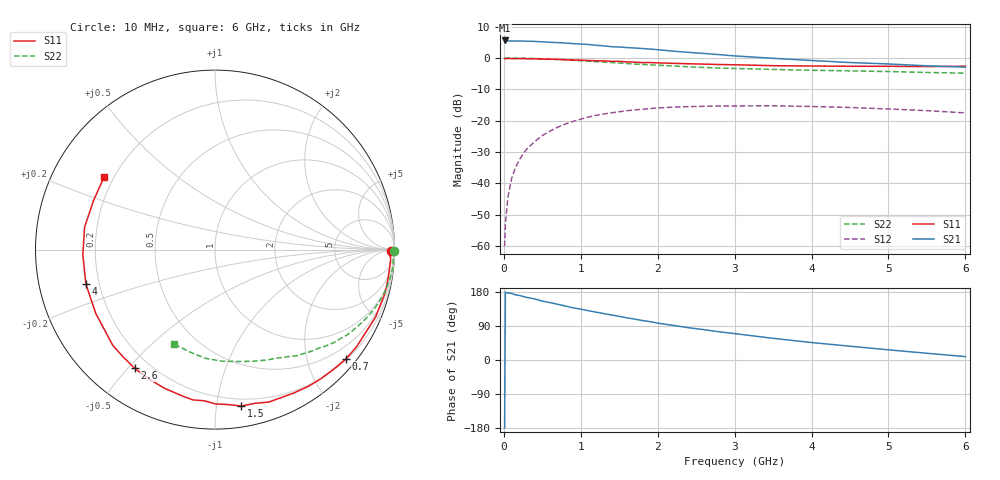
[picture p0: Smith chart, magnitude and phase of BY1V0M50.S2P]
! SIEMENS Small Signal Semiconductors
! BFY420
! Si NPN RF SIEGET Grounded Emitter Transistor in MICRO-X
! VCE = 1 V  IC = 0.5 mA
! Common Emitter S-Parameters:  October  1996
# GHz  S  MA  R  50
!  f  S11  S21  S12  S22
! GHz  MAG  ANG  MAG  ANG  MAG  ANG  MAG  ANG
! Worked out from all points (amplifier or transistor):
!   36 points, 10 MHz to 6 GHz, reference 50 ohm
!   highest |S21| = 5.6 dB at 10 MHz (marker M1)
!   |S21| within 3 dB of that: start of sweep to 2.022 GHz
!   unconditionally stable (mu >= 1): 4.728 GHz to end of sweep
!   at 250 MHz: K = 0.02, MSG = 18.0 dB, |S12| = -30.6 dB
!   at 1.4 GHz: K = 0.22, MSG = 10.5 dB, |S12| = -17.5 dB
!   at 6 GHz: K = 1.37, MAG = 3.7 dB, |S12| = -17.5 dB
!   S11 on the Smith chart (normalised r, x): 10 MHz: 80, -43; 700 MHz: 0.22, -2.75; 1.5 GHz: 0.15, -1.17; 2.6 GHz: 0.14, -0.52; 4 GHz: 0.15, -0.13; 6 GHz: 0.16, +0.29
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0.01  0.9808 -0.6  1.903 -179.2  0.001 101.0  0.9995 -0.4
0.02  0.9704 -1.3  1.888 178.8  0.0022 79.4  0.9999 -0.6
0.05  0.98 -2.8  1.874 177.1  0.0057 87.3  0.9986 -1.5
0.1  0.9783 -5.9  1.865 175.7  0.0119 88.1  0.9941 -3.0
0.15  0.9773 -8.5  1.863 172.0  0.0177 83.5  0.9951 -4.6
0.2  0.9777 -11.6  1.865 170.5  0.0237 82.2  0.9954 -6.0
0.3  0.9731 -17.3  1.849 165.2  0.0355 78.9  0.9887 -9.1
0.4  0.9701 -23.0  1.838 161.2  0.0465 75.0  0.9808 -12.1
0.5  0.9583 -28.7  1.806 155.4  0.0581 71.2  0.971 -15.0
0.7  0.9507 -39.7  1.76 147.0  0.0787 64.1  0.9463 -20.5
0.9  0.9304 -50.6  1.695 137.7  0.0977 56.8  0.9176 -25.7
1.1  0.912 -61.0  1.64 130.1  0.1142 50.3  0.8886 -30.7
1.5  0.884 -80.4  1.495 115.2  0.1391 37.9  0.8309 -39.3
1.8  0.8443 -94.1  1.416 104.1  0.1521 30.1  0.7894 -44.9
2.2  0.8219 -110.2  1.285 91.4  0.1647 20.3  0.7485 -52.1
2.6  0.7983 -124.1  1.18 80.1  0.1695 12.6  0.7074 -58.2
3  0.7799 -137.0  1.079 69.6  0.1721 5.5  0.6814 -64.4
3.5  0.7536 -151.7  0.988 57.2  0.1728 -2.0  0.6572 -71.2
4  0.7447 -165.0  0.912 46.1  0.1685 -8.6  0.6361 -78.6
4.5  0.7369 -177.7  0.846 36.4  0.1626 -14.3  0.6231 -86.2
5.5  0.7299 157.9  0.75 17.8  0.1447 -22.7  0.5874 -103.8
6  0.7386 146.8  0.715 9.0  0.1332 -24.9  0.5728 -113.6
